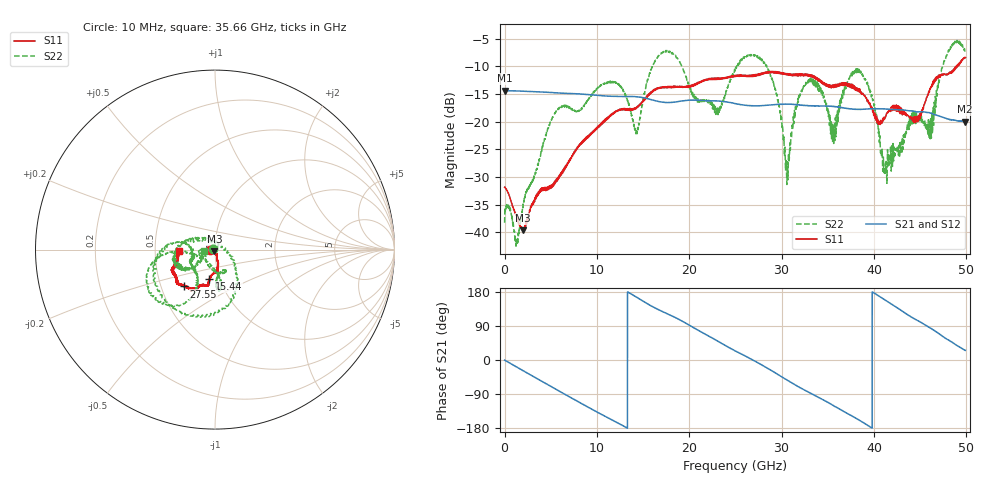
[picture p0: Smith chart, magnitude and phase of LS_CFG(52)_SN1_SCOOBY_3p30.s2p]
!Keysight Technologies,N5245B,MY58422026,A.13.80.08
!Date: Thursday, March 19, 2020 23:43:11
!Correction: S11(Full 2 Port(1,2))
!S21(Full 2 Port(1,2))
!S12(Full 2 Port(1,2))
!S22(Full 2 Port(1,2))
!S2P File: Measurements: S11, S21, S12, S22:
# Hz S DB R 50.0
!freq dBS11 angS11 dBS21 angS21 dBS12 angS12 dBS22 angS22
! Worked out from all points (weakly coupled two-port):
!   4991 points, 10 MHz to 49.91 GHz, reference 50 ohm
!   highest |S21| = -14.37 dB at 10 MHz (marker M1); lowest = -20.0 dB at 49.82 GHz (marker M2)
!   lowest |S11| = -39.6 dB at 2.02 GHz (marker M3), VSWR 1.02, Z = 49.6 - j0.982 ohm
!   |S11| at or under -10 dB: start of sweep to 48.9 GHz; 48.93138 GHz to 48.99547 GHz (64.09 MHz wide, 0.131 % of centre)
!   |S22| runs from -42.5 to -5.3 dB; largest |S21 - S12| = 0.0019
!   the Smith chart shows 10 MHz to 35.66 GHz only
!   S11 on the Smith chart (normalised r, x): 10 MHz: 0.95, -0.01; 15.44 GHz: 0.89, -0.30; 27.55 GHz: 0.65, -0.29; 35.66 GHz: 0.66, -0.01
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1e7  -31.84 -173.8  -14.37 -0.3  -14.35 -0.3  -38.24 175.3
1.34e9  -37.30 -152.0  -14.45 -18.9  -14.44 -18.8  -41.89 -44.4
2.02e9  -39.60 -109.2  -14.49 -28.4  -14.48 -28.3  -34.95 41.7
5.38e9  -30.92 -75.2  -14.76 -74.8  -14.75 -74.8  -18.71 -95.4
8.33e9  -23.99 -77.5  -15.01 -114.8  -15.00 -114.7  -17.66 -77.0
1.203e10  -18.20 -83.5  -15.44 -163.2  -15.43 -163.1  -13.01 -83.4
1.431e10  -17.44 -93.5  -15.49 165.6  -15.48 165.7  -21.97 -128.5
1.544e10  -15.59 -100.7  -15.84 149.0  -15.83 149.0  -12.82 -177.7
1.665e10  -14.00 -101.2  -16.33 133.1  -16.32 133.2  -8.20 -162.3
2.299e10  -12.31 -115.1  -16.24 51.2  -16.24 51.4  -18.47 -166.5
2.496e10  -11.80 -121.0  -16.69 24.4  -16.68 24.6  -10.73 -177.9
2.755e10  -11.43 -130.0  -17.12 -8.7  -17.12 -8.5  -8.48 -101.2
2.933e10  -10.95 -139.4  -16.89 -34.1  -16.90 -33.9  -14.17 -50.9
3.063e10  -11.40 -144.3  -16.83 -53.5  -16.83 -53.2  -27.65 65.7
3.328e10  -11.74 -157.1  -17.12 -89.5  -17.12 -89.1  -12.47 -160.3
3.566e10  -13.78 -178.0  -17.23 -120.7  -17.16 -120.3  -23.77 176.0
3.839e10  -14.51 171.0  -17.78 -158.4  -17.72 -158.7  -10.61 -160.9
4.16e10  -17.95 104.4  -17.74 152.3  -17.76 152.3  -25.76 111.3
4.675e10  -11.96 8.2  -18.80 74.5  -18.82 74.7  -14.88 -139.1
4.841e10  -11.04 -6.0  -19.69 47.8  -19.73 47.9  -6.21 -62.9
4.982e10  -8.47 -15.7  -20.00 26.3  -20.01 26.5  -6.90 -12.6
4.991e10  -8.40 -14.9  -19.98 25.3  -20.01 25.3  -7.49 -12.9
